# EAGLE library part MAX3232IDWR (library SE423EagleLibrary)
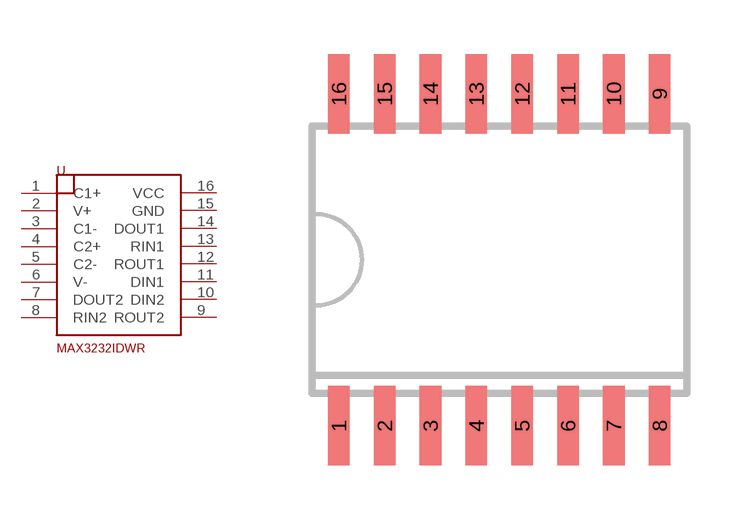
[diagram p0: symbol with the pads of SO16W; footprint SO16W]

Designator prefix U

## MAX3232IDWR  [SO16W]
1  C1+
2  V+
3  C1-
4  C2+
5  C2-
6  V-
7  DOUT2
8  RIN2
9  ROUT2
10  DIN2
11  DIN1
12  ROUT1
13  RIN1
14  DOUT1
15  GND
16  VCC

## Footprint SO16W (pad centres in mm)
SMALL OUTLINE INTEGRATED CIRCUIT wide body 7.5 mm/JEDEC MS-013AA
smd 0.6 x 2.2: 1 -4.445,-4.6; 2 -3.175,-4.6; 3 -1.905,-4.6; 4 -0.635,-4.6; 5 0.635,-4.6; 6 1.905,-4.6; 7 3.175,-4.6; 8 4.445,-4.6; 9 4.445,4.6; 10 3.175,4.6; 11 1.905,4.6; 12 0.635,4.6; 13 -0.635,4.6; 14 -1.905,4.6; 15 -3.175,4.6; 16 -4.445,4.6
